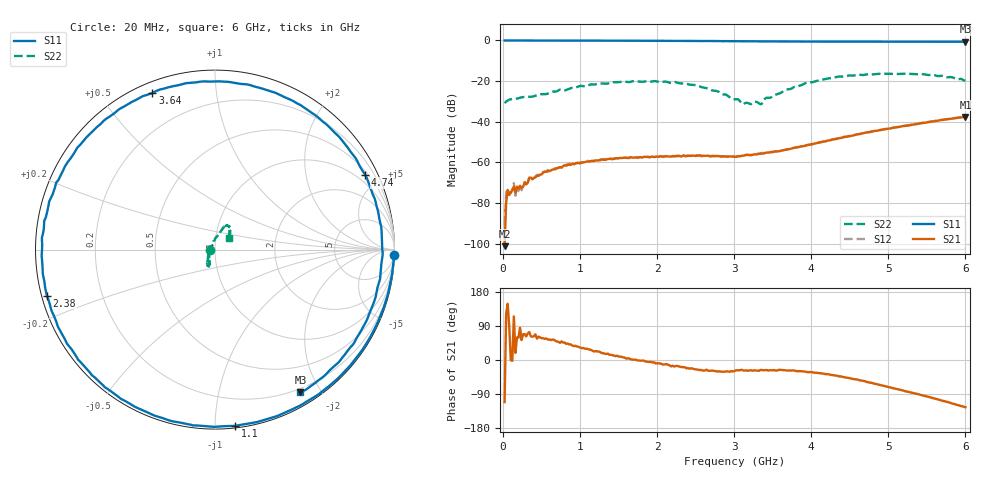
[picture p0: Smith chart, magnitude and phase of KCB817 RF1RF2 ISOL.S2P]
!Agilent Technologies,E5071B,JP1KK00126,A.08.11
!Date: Mon Apr 22 13:19:31 2013
!Data & Calibration Information:
!Freq	S11:SOLT2(ON)	S21:SOLT2(ON)	S12:SOLT2(ON)	S22:SOLT2(ON)
# Hz S dB R 50
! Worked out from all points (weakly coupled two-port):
!   300 points, 20 MHz to 6 GHz, reference 50 ohm
!   highest |S21| = -37.61 dB at 6 GHz (marker M1); lowest = -101.2 dB at 20 MHz (marker M2)
!   lowest |S11| = -0.7 dB at 6 GHz (marker M3), VSWR 26.34, Z = 7.76 - j87.6 ohm
!   |S11| at or under -10 dB: nowhere
!   |S22| runs from -31.4 to -16.3 dB; largest |S21 - S12| = 0.00024
!   S11 on the Smith chart (normalised r, x): 20 MHz: 9, -71; 1.1 GHz: 0.01, -1.12; 2.38 GHz: 0.02, -0.13; 3.64 GHz: 0.05, +0.68; 4.74 GHz: 0.63, +4.16; 6 GHz: 0.16, -1.75
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2e7  -0.03 -1.6  -101.19 -111.0  -90.64 -166.9  -30.86 -173.7
4e7  -0.02 -3.2  -79.66 122.9  -74.57 124.3  -30.06 -172.4
6e7  -0.03 -4.7  -73.53 148.3  -73.36 144.3  -29.55 -171.1
1e8  -0.04 -8.1  -74.79 -0.5  -75.01 -8.1  -28.94 -166.3
1.4e8  -0.05 -11.0  -71.96 114.9  -70.14 126.4  -28.76 -162.4
1.6e8  -0.05 -12.6  -74.99 18.8  -76.42 29.7  -28.72 -161.0
1.8e8  -0.04 -14.3  -71.89 59.3  -71.40 57.1  -28.62 -160.7
2.4e8  -0.05 -18.8  -72.63 52.6  -73.67 48.5  -28.00 -156.2
3.6e8  -0.07 -28.1  -67.49 62.6  -67.37 60.0  -27.70 -145.2
1.02e9  -0.10 -76.9  -60.20 31.3  -59.80 31.5  -22.40 -113.2
1.1e9  -0.10 -83.5  -59.51 28.9  -59.21 27.6  -22.24 -114.6
1.52e9  -0.15 -110.9  -57.78 9.1  -57.95 8.2  -20.43 -108.9
2.02e9  -0.20 -141.7  -57.27 -8.6  -57.24 -9.3  -20.38 -113.1
2.38e9  -0.26 -164.7  -56.93 -22.1  -56.70 -21.4  -21.31 -120.1
3.02e9  -0.40 156.2  -57.26 -27.5  -57.31 -26.9  -28.91 -161.8
3.34e9  -0.46 133.9  -55.74 -26.2  -55.59 -27.6  -31.39 133.7
3.64e9  -0.54 111.8  -53.99 -26.5  -54.01 -28.2  -24.85 90.3
4.02e9  -0.58 83.0  -51.00 -32.9  -50.85 -32.7  -20.52 75.7
4.74e9  -0.58 26.5  -45.18 -58.4  -45.01 -59.2  -16.61 65.0
5.02e9  -0.59 6.5  -43.33 -72.0  -43.19 -72.6  -16.35 62.3
5.5e9  -0.61 -26.5  -40.31 -96.4  -40.19 -96.4  -16.98 55.3
6e9  -0.66 -59.1  -37.61 -124.6  -37.49 -124.8  -19.95 40.9
